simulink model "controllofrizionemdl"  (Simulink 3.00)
settings: Solver=ode45  StartTime=0.0  StopTime=10.0  RelTol=1e-5
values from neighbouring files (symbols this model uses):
  A = 4*(cm^2)    (= 0.0004)    [controllofrizione.m]
  b = 0.25*10^2*N*sec/m    (= 25)    [controllofrizione.m]
  Cm = 1*10^(-10)*m^3/Pa    (= 1e-10)    [controllofrizione.m]
  Km = 0.8*10^4*N/m    (= 8000)    [controllofrizione.m]
  Krc = 1    [controllofrizione.m]
  Kv = 3*10^(-9)*m^3/(sec*Pa)    (= 3e-09)    [controllofrizione.m]
  mp = 0.3*Kg    (= 0.3)    [controllofrizione.m]
  P10 = 0*bar    (= 0)    [controllofrizione.m]
  tau1 = 0    [controllofrizione.m]
  tau2 = 0    [controllofrizione.m]
  x0 = 0*cm    (= 0)    [controllofrizione.m]
libraries: simulink3 x1

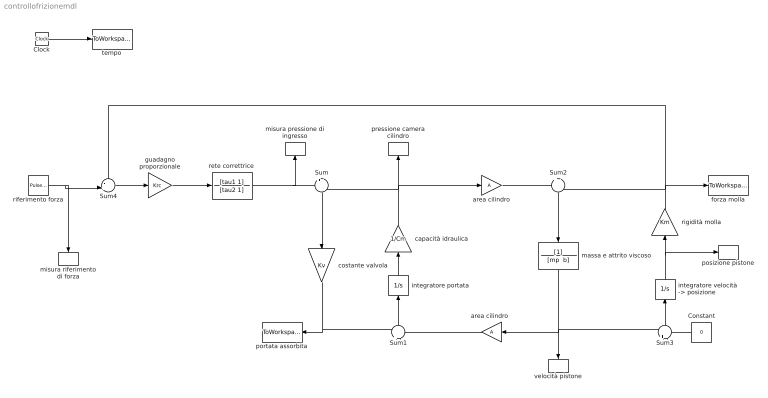
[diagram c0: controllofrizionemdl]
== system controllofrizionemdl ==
  Clock : Clock
  Constant : Constant  Orientation=left  Value=0
  Sum : Sum  Orientation=down  Inputs=+-  SaturateOnIntegerOverflow=on
  Sum1 : Sum  Orientation=up  Inputs=+-  SaturateOnIntegerOverflow=on
  Sum2 : Sum  Orientation=down  Inputs=+-  SaturateOnIntegerOverflow=on
  Sum3 : Sum  Orientation=up  Inputs=+-  SaturateOnIntegerOverflow=on
  Sum4 : Sum  Inputs=-+|  SaturateOnIntegerOverflow=on
  area cilindro : Gain  Gain=A  SaturateOnIntegerOverflow=on
  "area cilindro  " : Gain  Orientation=left  Gain=A  SaturateOnIntegerOverflow=on
  capacità idraulica : Gain  Orientation=up  Gain=1/Cm  SaturateOnIntegerOverflow=on
  costante valvola : Gain  Orientation=down  Gain=Kv  SaturateOnIntegerOverflow=on
  forza molla : ToWorkspace  VariableName=Fm  SampleTime=-1  SaveFormat=Matrix
  guadagno proporzionale : Gain  Gain=Krc  SaturateOnIntegerOverflow=on
  integratore portata : Integrator  Orientation=up  ExternalReset=none  InitialConditionSource=internal  InitialCondition=P10  LimitOutput=off  UpperSaturationLimit=inf  LowerSaturationLimit=-inf  ShowSaturationPort=off  ShowStatePort=off  AbsoluteTolerance=auto
  "integratore velocità -> posizione" : Integrator  Orientation=up  ExternalReset=none  InitialConditionSource=internal  InitialCondition=x0  LimitOutput=off  UpperSaturationLimit=inf  LowerSaturationLimit=-inf  ShowSaturationPort=off  ShowStatePort=off  AbsoluteTolerance=auto
  massa e attrito viscoso : TransferFcn  Orientation=down  Numerator=[1]  Denominator="[mp  b]"
  misura pressione di ingresso : ToWorkspace  VariableName=P  SampleTime=-1  SaveFormat=Matrix
  misura riferimento di forza : ToWorkspace  VariableName=Fmr  SampleTime=-1  SaveFormat=Matrix
  portata assorbita : ToWorkspace  VariableName=Q  SampleTime=-1  SaveFormat=Matrix
  posizione pistone : ToWorkspace  VariableName=x  SampleTime=-1  SaveFormat=Matrix
  pressione camera cilindro : ToWorkspace  VariableName=P1  SampleTime=-1  SaveFormat=Matrix
  rete correttrice : TransferFcn  Numerator=[tau1 1]  Denominator=[tau2 1]
  riferimento forza : simulink3/Sources/Pulse Generator  period=Tr  duty=DCr  amplitude=Fmr  start=0
  rigidità molla : Gain  Orientation=up  Gain=Km  SaturateOnIntegerOverflow=on
  tempo : ToWorkspace  VariableName=t  SampleTime=-1  SaveFormat=Matrix
  velocità pistone : ToWorkspace  VariableName=xdot  SampleTime=-1  SaveFormat=Matrix
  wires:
  "integratore velocità -> posizione"/1 -> rigidità molla/1, posizione pistone/1
  Sum3/1 -> "integratore velocità -> posizione"/1
  Sum2/1 -> massa e attrito viscoso/1
  rigidità molla/1 -> Sum2/2, forza molla/1, Sum4/1
  massa e attrito viscoso/1 -> Sum3/1, "area cilindro  "/1, velocità pistone/1
  Constant/1 -> Sum3/2
  Sum1/1 -> integratore portata/1
  area cilindro/1 -> Sum2/1
  "area cilindro  "/1 -> Sum1/2
  capacità idraulica/1 -> area cilindro/1, pressione camera cilindro/1, Sum/2
  integratore portata/1 -> capacità idraulica/1
  costante valvola/1 -> Sum1/1, portata assorbita/1
  Sum/1 -> costante valvola/1
  guadagno proporzionale/1 -> rete correttrice/1
  rete correttrice/1 -> Sum/1, misura pressione di ingresso/1
  riferimento forza/1 -> Sum4/2, misura riferimento di forza/1
  Clock/1 -> tempo/1
  Sum4/1 -> guadagno proporzionale/1
